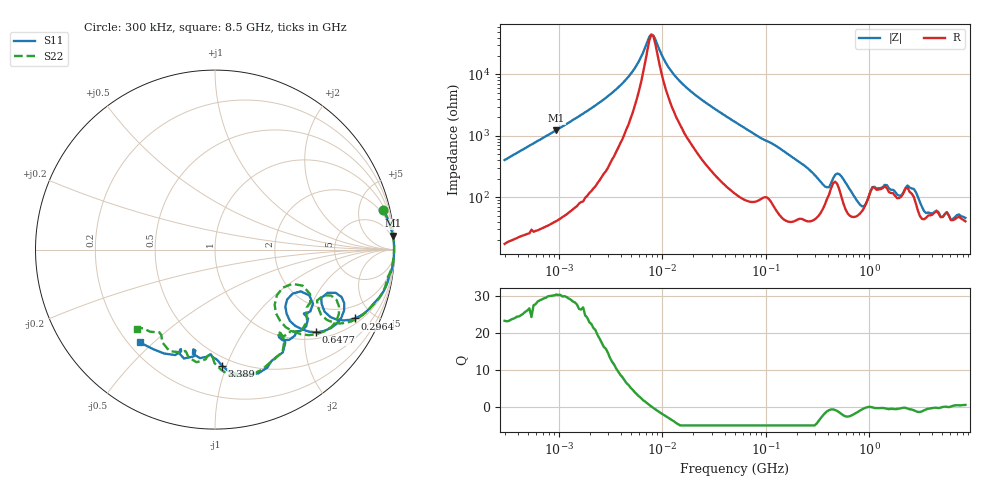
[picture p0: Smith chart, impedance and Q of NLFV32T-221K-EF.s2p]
! S-parameter Generated by TDK Corporation
! Copyright(C) 2015 TDK Corporation.
! All Rights Reserved.
! TDK P/N: NLFV32T-221K-EF (Inductors)
! Property: L=220uH at 796kHz
! Size(LxWxT): 3.2x2.5x2.2mm, 0.126x0.098x0.087inches
! Model Type: s2p (Touchstone File Format Version 1.0)
! Frequency: DC=Yes Start=0.3MHz Stop=8500MHz 225points Log-sweep
! Note:
! Model Generated on Jun. 23, 2015
! Hash(MD5):
! Port Assignments:
!  1 ---@@@--- 2
! Applicable Conditions:
!  Temperature = 25 degC
!  DC Bias Current = 0 A
!  Small Signal Operation
! Terms and conditions regarding TDK Simulation Models
! (1)This simulation model is being provided solely for informational purposes. Please refer to the specifications of the products in terms of detailed characteristics of such products.
! (2)In no event shall TDK Corporation of any of its subsidiaries be liable for any loss or damage arising, directly or indirectly,
!  From any information contained in this simulation model, including, but not limited to loss or damages arising from any inaccuracies, omissions or errors in connection with such information.
! (3)Any and all copyrights on this simulation model are owned by TDK Corporation.
!  Duplication or redistribution of this simulation model without prior written permission from TDK Corporation is prohibited.
! (4)This simulation model is subject to any modification or change without any prior notice.
! (5)Neither TDK Corporation nor any of its subsidiaries shall make any warranty, express or implied,
!  Including but not limited to the correctness, implied warranties of merchantability and fitness for a particular purpose with respect to this simulation models.
! (6)The use of this simulation model shall be deemed to have consented to the terms and conditions hereof.
# MHz S MA R 50
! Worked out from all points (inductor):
!   224 points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, 300 kHz to 8.5 GHz, reference 50 ohm
!   read as one part in series: L = 212 uH near 314.1 kHz
!   highest Q = 30.3 at 946.8 kHz (marker M1), where L = 208 uH
!   self-resonance near 7.846 MHz
!   S11 on the Smith chart (normalised r, x): 300 kHz: 1.41, +8.27; 296.4 MHz: 1.26, -3.91; 647.7 MHz: 1.17, -2.29; 3.389 GHz: 0.43, -0.96; 8.5 GHz: 0.24, -0.45
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0.3  0.9613 13.4  0.2381 -74.1  0.2411 -74.3  0.9604 13.4
0.9467989  0.9938 4.5  0.0802 -83.7  0.08062 -84.0  0.9943 4.4
1.72111  0.9972 2.4  0.04334 -85.5  0.04351 -85.9  0.9979 2.3
4.519427  0.9981 0.6  0.01182 -80.7  0.01184 -81.1  0.9982 0.4
7.846373  0.9979 -0.2  0.002225 -7.9  0.002226 -8.1  0.9977 -0.3
9.430415  0.9978 -0.4  0.003996 54.3  0.003989 54.2  0.9976 -0.5
15.63691  0.9975 -1.1  0.01409 78.3  0.0141 78.0  0.9971 -1.3
51.67171  0.9948 -4.4  0.06036 81.6  0.0604 81.3  0.9921 -4.8
283.1228  0.8856 -24.9  0.3437 55.1  0.3439 54.9  0.8757 -26.3
296.4424  0.8679 -26.2  0.3636 52.5  0.3639 52.3  0.858 -27.8
390.6008  0.6678 -27.1  0.4382 23.8  0.4386 23.5  0.6552 -29.0
448.3627  0.7138 -19.7  0.3358 15.1  0.3361 14.7  0.6955 -21.6
647.669  0.7285 -39.2  0.4848 29.3  0.4851 29.0  0.7069 -42.4
815.0429  0.5373 -41.9  0.5857 7.2  0.5863 6.9  0.4915 -46.3
979.5854  0.5316 -26.0  0.4944 -14.5  0.494 -15.0  0.4714 -23.9
1073.923  0.6239 -28.9  0.3929 -13.7  0.3923 -13.8  0.5854 -25.1
1551.304  0.657 -43.7  0.392 -6.1  0.3924 -6.7  0.6373 -45.9
2346.313  0.6861 -56.6  0.3389 -21.2  0.3392 -21.5  0.6816 -56.5
2952.659  0.7223 -75.7  0.4165 -12.7  0.4174 -13.3  0.7182 -79.1
3389.298  0.6473 -86.6  0.5048 -24.9  0.5044 -25.0  0.6321 -90.3
7072.242  0.598 -108.5  0.41 -82.7  0.4117 -83.4  0.5659 -125.5
8500  0.6655 -129.0  0.3354 -99.0  0.3349 -98.3  0.622 -134.5
